PROGRAM MAIN
VAR
	BoolTest AT %MB0:BOOL;
	IntTest AT %MB2:INT;
	UintTest AT %QB0:UINT;
	StringTest:STRING:='This is tc3,do you copy?';
	RealTest AT %MB4:REAL;
	LrealTest AT %QB4:LREAL;
	ArrayTest AT %MB8:ARRAY[0..4] OF LREAL;
	writeonly AT %MB100:INT;

	
END_VAR

IF IntTest < 32767 THEN
IntTest := IntTest +1;
ELSE
	IntTest := -32768;
END_IF

END_PROGRAM
